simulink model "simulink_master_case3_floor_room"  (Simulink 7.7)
settings: Solver=ode23s  StartTime=0.0  StopTime=72000  FixedStep=48  RelTol=1e-6
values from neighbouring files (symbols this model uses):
  Tfmax = 298    [model_master_simulink_floor.m]    (also in model_master_simulink_PI_tuning.m; model_master_simulink_storing_floorroom.m)
  Tfmin = 293    [model_master_simulink_floor.m]    (also in model_master_simulink_PI_tuning.m; model_master_simulink_storing_floorroom.m)
  To = 273+0    (= 273)    [model_master_simulink_floor.m]    (also in model_master_simulink_PI_tuning.m; model_master_simulink_storing_floorroom.m; sfunctionmodel.m = u(3); equations.m = d(1))
  Trmax = 298    [model_master_simulink_floor.m]    (also in model_master_simulink_PI_tuning.m; model_master_simulink_storing_floorroom.m)
  Trmin = 292    [model_master_simulink_floor.m]    (also in model_master_simulink_PI_tuning.m; model_master_simulink_storing_floorroom.m)
libraries: simulink x2

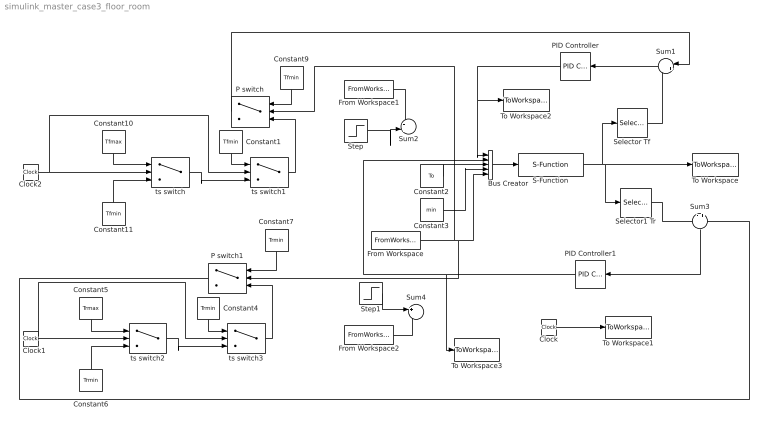
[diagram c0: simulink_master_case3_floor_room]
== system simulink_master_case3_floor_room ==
  Bus Creator : BusCreator  Inputs=5
  Clock : Clock
  Clock1 : Clock
  Clock2 : Clock
  Constant1 : Constant  Value=Tfmin
  Constant10 : Constant  Value=Tfmax
  Constant11 : Constant  Value=Tfmin
  Constant2 : Constant  Value=To
  Constant3 : Constant  Value=min
  Constant4 : Constant  Value=Trmin
  Constant5 : Constant  Value=Trmax
  Constant6 : Constant  Value=Trmin
  Constant7 : Constant  Value=Trmin
  Constant9 : Constant  Value=Tfmin
  From Workspace : FromWorkspace  VariableName=var  SampleTime=0  Interpolate=off  OutputAfterFinalValue=Holding final value
  From Workspace1 : FromWorkspace  VariableName=varqhf  SampleTime=0
  From Workspace2 : FromWorkspace  VariableName=varqhr  SampleTime=0
  P switch : Switch  Threshold=0.8/(60*60)
  P switch1 : Switch  Threshold=0.8/(60*60)
  PID Controller : simulink/Continuous/PID Controller  SystemSampleTime=-1  Controller=PI  TimeDomain=Continuous-time  SampleTime=1  IntegratorMethod=Forward Euler  FilterMethod=Forward Euler  Form=Parallel  P=127.7  I=3192.5*0.0001  D=0  N=100  InitialConditionSource=internal  InitialConditionForIntegrator=0  InitialConditionForFilter=0  ExternalReset=none  LimitOutput=on  UpperSaturationLimit=2.5  LowerSaturationLimit=0  LinearizeAsGain=off  AntiWindupMode=clamping  Kb=1  TrackingMode=off  Kt=1  PParamMin=[]  PParamMax=[]  IParamMin=[]  IParamMax=[]  DParamMin=[]  DParamMax=[]  NParamMin=[]  NParamMax=[]  KbParamMin=[]  KbParamMax=[]  KtParamMin=[]  KtParamMax=[]  POutMin=[]  POutMax=[]  IOutMin=[]  IOutMax=[]  DOutMin=[]  DOutMax=[]  NOutMin=[]  NOutMax=[]  KbOutMin=[]  KbOutMax=[]  KtOutMin=[]  KtOutMax=[]  IntegratorOutMin=[]  IntegratorOutMax=[]  FilterOutMin=[]  FilterOutMax=[]  SumOutMin=[]  SumOutMax=[]  SumI1OutMin=[]  SumI1OutMax=[]  SumI2OutMin=[]  SumI2OutMax=[]  SumI3OutMin=[]  SumI3OutMax=[]  SumDOutMin=[]  SumDOutMax=[]  SaturationOutMin=[]  SaturationOutMax=[]  IntegratorContinuousStateAttributes=''  IntegratorStateMustResolveToSignalObject=off  IntegratorRTWStateStorageClass=Auto  FilterContinuousStateAttributes=''  FilterStateMustResolveToSignalObject=off  FilterRTWStateStorageClass=Auto
  PID Controller1 : simulink/Continuous/PID Controller  SystemSampleTime=-1  Controller=PI  TimeDomain=Continuous-time  SampleTime=1  IntegratorMethod=Forward Euler  FilterMethod=Forward Euler  Form=Parallel  P=249.7  I=6242.5*0.1  D=0  N=100  InitialConditionSource=internal  InitialConditionForIntegrator=0  InitialConditionForFilter=0  ExternalReset=none  LimitOutput=on  UpperSaturationLimit=2  LowerSaturationLimit=0  LinearizeAsGain=off  AntiWindupMode=clamping  Kb=1  TrackingMode=off  Kt=1  PParamMin=[]  PParamMax=[]  IParamMin=[]  IParamMax=[]  DParamMin=[]  DParamMax=[]  NParamMin=[]  NParamMax=[]  KbParamMin=[]  KbParamMax=[]  KtParamMin=[]  KtParamMax=[]  POutMin=[]  POutMax=[]  IOutMin=[]  IOutMax=[]  DOutMin=[]  DOutMax=[]  NOutMin=[]  NOutMax=[]  KbOutMin=[]  KbOutMax=[]  KtOutMin=[]  KtOutMax=[]  IntegratorOutMin=[]  IntegratorOutMax=[]  FilterOutMin=[]  FilterOutMax=[]  SumOutMin=[]  SumOutMax=[]  SumI1OutMin=[]  SumI1OutMax=[]  SumI2OutMin=[]  SumI2OutMax=[]  SumI3OutMin=[]  SumI3OutMax=[]  SumDOutMin=[]  SumDOutMax=[]  SaturationOutMin=[]  SaturationOutMax=[]  IntegratorContinuousStateAttributes=''  IntegratorStateMustResolveToSignalObject=off  IntegratorRTWStateStorageClass=Auto  FilterContinuousStateAttributes=''  FilterStateMustResolveToSignalObject=off  FilterRTWStateStorageClass=Auto
  S-Function : S-Function  FunctionName=sfunctionmodel  Parameters=init, par,var  EnableBusSupport=off
  Selector Tf : Selector  InputPortWidth=3  IndexOptions=Index vector (dialog)  Indices=1  OutputSizes=1
  Selector1 Tr : Selector  InputPortWidth=3  IndexOptions=Index vector (dialog)  Indices=2  OutputSizes=1
  Step : Step  Time=10*60*60  After=5  SampleTime=0
  Step1 : Step  Time=10*60*60  After=4  SampleTime=0
  Sum1 : Sum  Inputs=|+-
  Sum2 : Sum  Inputs=-+
  Sum3 : Sum  Inputs=-+
  Sum4 : Sum  Inputs=+-
  To Workspace : ToWorkspace  VariableName=simout  SampleTime=-1  SaveFormat=Array
  To Workspace1 : ToWorkspace  VariableName=time  SampleTime=-1  SaveFormat=Array
  To Workspace2 : ToWorkspace  VariableName=qhf_out  SampleTime=-1  SaveFormat=Array
  To Workspace3 : ToWorkspace  VariableName=qhr_out  SampleTime=-1  SaveFormat=Array
  ts switch : Switch  ZeroCross=off
  ts switch1 : Switch  Threshold=3*60*60  ZeroCross=off
  ts switch2 : Switch  Threshold=2.2*60*60  ZeroCross=off
  ts switch3 : Switch  Threshold=3*60*60  ZeroCross=off
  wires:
  Constant3/1 -> Bus Creator/4
  Bus Creator/1 -> S-Function/1
  S-Function/1 -> To Workspace/1, Selector1 Tr/1, Selector Tf/1
  Selector1 Tr/1 -> Sum3/1
  Sum3/1 -> PID Controller1/1
  Constant2/1 -> Bus Creator/3
  Selector Tf/1 -> Sum1/2
  Sum1/1 -> PID Controller/1
  From Workspace/1 -> P switch/2, Bus Creator/5, P switch1/2
  Step/1 -> Sum2/2
  From Workspace1/1 -> Sum2/1
  PID Controller/1 -> To Workspace2/1, Bus Creator/1
  Step1/1 -> Sum4/1
  From Workspace2/1 -> Sum4/2
  PID Controller1/1 -> To Workspace3/1, Bus Creator/2
  Constant9/1 -> P switch/1
  Constant10/1 -> ts switch/1
  Constant11/1 -> ts switch/3
  Clock2/1 -> ts switch1/2, ts switch/2
  P switch/1 -> Sum1/1
  Clock/1 -> To Workspace1/1
  Constant1/1 -> ts switch1/1
  ts switch1/1 -> P switch/3
  ts switch/1 -> ts switch1/3
  Constant7/1 -> P switch1/1
  Constant5/1 -> ts switch2/1
  Constant6/1 -> ts switch2/3
  Clock1/1 -> ts switch3/2, ts switch2/2
  Constant4/1 -> ts switch3/1
  ts switch3/1 -> P switch1/3
  ts switch2/1 -> ts switch3/3
  P switch1/1 -> Sum3/2
